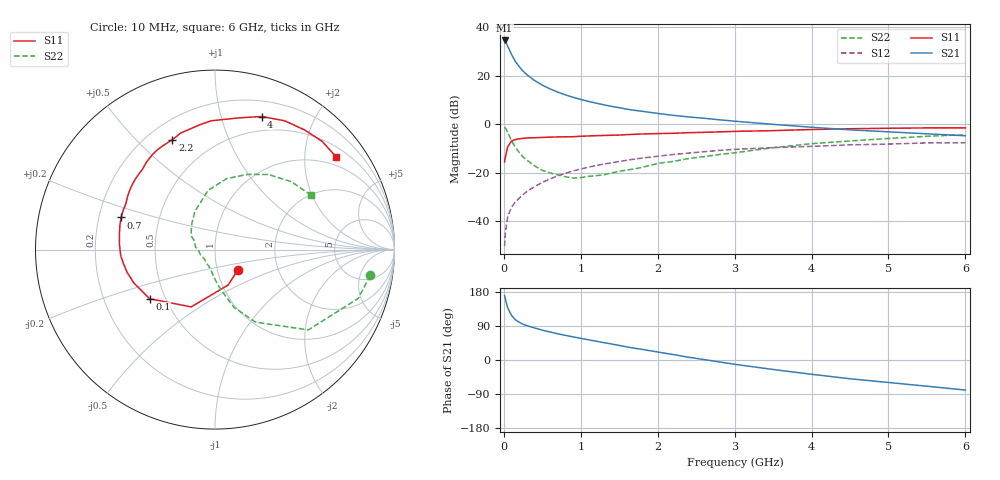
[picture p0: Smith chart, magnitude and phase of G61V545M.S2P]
! SIEMENS Small Signal Semiconductors
! BFG193
! Si NPN RF Bipolar Junction Transistor in SOT223
! VCE = 1.5 V  IC = 45 mA
! Common Emitter S-Parameters:  August  1996
# GHz  S  MA  R  50
!  f  S11  S21  S12  S22
! GHz  MAG  ANG  MAG  ANG  MAG  ANG  MAG  ANG
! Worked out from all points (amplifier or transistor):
!   36 points, 10 MHz to 6 GHz, reference 50 ohm
!   highest |S21| = 34.6 dB at 10 MHz (marker M1)
!   |S21| within 3 dB of that: start of sweep to 60.22 MHz
!   unconditionally stable (mu >= 1): 369.6 MHz to 2.687 GHz
!   at 250 MHz: K = 0.94, MSG = 25.5 dB, |S12| = -28.9 dB
!   at 1.4 GHz: K = 1.07, MAG = 10.0 dB, |S12| = -15.8 dB
!   at 6 GHz: K = 0.95, MSG = 1.5 dB, |S12| = -7.6 dB
!   S11 on the Smith chart (normalised r, x): 10 MHz: 1.26, -0.29; 100 MHz: 0.41, -0.28; 700 MHz: 0.30, +0.15; 2.2 GHz: 0.30, +0.64; 4 GHz: 0.35, +1.35; 6 GHz: 0.75, +2.78
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0.01  0.1698 -40.9  53.77 169.7  0.0031 79.7  0.8773 -9.4
0.02  0.2106 -69.6  51.4 160.5  0.0059 75.3  0.8432 -18.8
0.05  0.3458 -112.6  41.31 137.7  0.0126 65.5  0.6861 -40.7
0.1  0.4556 -143.1  27.68 117.7  0.0198 61.7  0.4623 -60.9
0.15  0.4881 -157.4  19.86 106.1  0.0252 61.6  0.3362 -72.0
0.2  0.5056 -165.4  15.51 99.6  0.0301 63.8  0.2643 -77.3
0.25  0.5168 -171.7  12.56 94.4  0.0358 64.4  0.2133 -83.0
0.3  0.5263 -176.3  10.59 90.6  0.0416 65.8  0.1838 -87.2
0.4  0.5331 176.8  8.04 84.5  0.0526 66.0  0.1399 -95.0
0.5  0.5398 170.7  6.444 78.8  0.0638 65.7  0.1134 -102.1
0.6  0.5469 165.5  5.404 74.0  0.0754 64.6  0.1001 -109.6
0.7  0.5531 161.1  4.645 69.2  0.087 63.5  0.0914 -119.0
0.9  0.5587 152.7  3.627 61.0  0.11 59.6  0.0785 -138.9
1.1  0.5792 145.1  2.982 53.3  0.1314 56.1  0.0851 -157.2
1.6  0.6171 128.6  2.063 34.6  0.183 44.4  0.1147 166.4
2.2  0.6568 111.2  1.542 14.4  0.2399 30.2  0.1727 139.8
2.8  0.7032 96.2  1.247 -5.0  0.2916 15.6  0.2402 117.9
3.5  0.7452 79.9  1.004 -25.0  0.333 -2.1  0.332 96.7
4  0.7857 70.7  0.875 -37.7  0.3533 -11.9  0.4008 80.7
4.5  0.8161 61.6  0.774 -49.5  0.3797 -22.0  0.4571 66.5
5.5  0.8485 45.3  0.641 -69.2  0.4167 -44.8  0.5694 41.6
6  0.8502 37.4  0.584 -79.3  0.4178 -57.8  0.6152 29.6
